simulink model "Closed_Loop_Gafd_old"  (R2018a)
settings: Solver=ode45  StartTime=0.0  StopTime=50  RelTol=1e-3  EnableMultiTasking=on
InitFcn:
  | init
StopFcn:
  | pl
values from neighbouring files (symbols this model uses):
  Cyb = -0.0245    [init.m]    (also in lqr_des.m)
  Cydel = [-0.24668,0.24668, 0.47413,-0.47413,0]/100    [init.m]    (also in lqr_des.m = [-0.24668,0.24668, 0.47413,-0.47413]/100)
  Cza = -0.073    [init.m]
  Czdel = [0.51664,0.51664,0.60478,0.60478,0.06]/100    [init.m]
  d2r = pi/180    (= 0.0174532925199)    [init.m]
  Mass = 198.32    [init.m]    (also in lqr_des.m)
  Qbar = 150    [init.m]    (also in lqr_des.m)
  r2d = 180/pi    (= 57.2957795131)    [init.m]    (also in pl.m)
  Sref = 79.069    [init.m]    (also in lqr_des.m)
  V0 = 822.8    [init.m]
undefined symbols (not defined in the file or in its folder): Abfp, Aema, Afla, Ardr, Avf, Bbfp, Bema, Bfla, Brdr, Bvf, Cbfp, Cema, Cfla, Crdr, Cvf, Dbfp, Dema, Dfla, Drdr, Dvf, K4axmix, Kf1, Kf2, Kf3, Kf4, Kf6, Kgl, Kgp, wd1, wd2, wd3, wd4, wd6, wd7, wn1, wn2, wn3, wn4, wn6, wn7, zd1, zd2, zd3, zd4, zd6, zd7, zn1, zn2, zn3, zn4, zn6, zn7

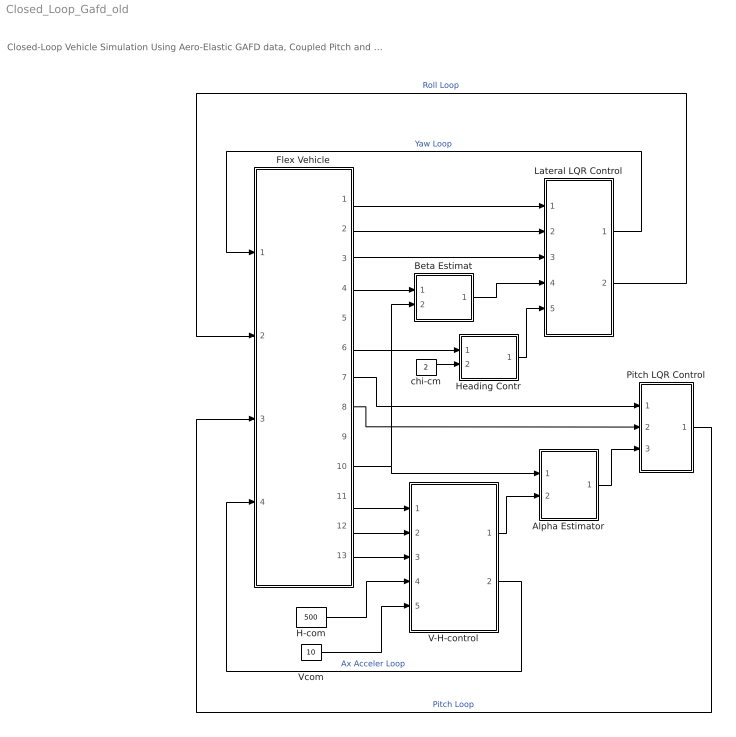
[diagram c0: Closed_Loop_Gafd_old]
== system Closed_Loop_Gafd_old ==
  note: Closed-Loop Vehicle Simulation Using Aero-Elastic GAFD data, Coupled Pitch and Lateral axes
  Alpha Estimator : Subsystem
  Beta Estimat : Subsystem
  Flex Vehicle : Subsystem
  H-com : Constant  Value=500
  Heading Contr : Subsystem
  Lateral LQR Control : Subsystem
  Pitch LQR Control : Subsystem
  V-H-control : Subsystem
  Vcom : Constant  Value=10
  chi-cm : Constant  Value=2
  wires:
  chi-cm/1 -> Heading Contr/2(chi-cmd)
  Flex Vehicle/2(p) -> Lateral LQR Control/2(p)
  Flex Vehicle/3(r) -> Lateral LQR Control/3(r)
  Flex Vehicle/1(phi) -> Lateral LQR Control/1(phi)
  Flex Vehicle/4(Ny) -> Beta Estimat/1(Ydd)
  Flex Vehicle/6("chi ") -> Heading Contr/1(chi)
  Flex Vehicle/12(Nz) -> V-H-control/2(Az)
  Flex Vehicle/13(dH) -> V-H-control/3(dH)
  Flex Vehicle/11(V-dot) -> V-H-control/1(Vdot)
  Flex Vehicle/10(delt) -> Alpha Estimator/1(delta), Beta Estimat/2(delta)
  Alpha Estimator/1(alphat) -> Pitch LQR Control/3(alfa)
  V-H-control/1(Zdd-com) -> Alpha Estimator/2(Zdd)
  Pitch LQR Control/1(elev) -> Flex Vehicle/3(ptch)  "Pitch Loop"
  Beta Estimat/1(bethat) -> Lateral LQR Control/4(bet)
  Lateral LQR Control/2(Rud) -> Flex Vehicle/2(yaw)  "Roll Loop"
  Lateral LQR Control/1(Ailer) -> Flex Vehicle/1(roll)  "Yaw Loop"
  V-H-control/2(Throtle) -> Flex Vehicle/4(Ax-cmd)  "Ax Acceler Loop"
  Flex Vehicle/8(q) -> Pitch LQR Control/2(q)
  Flex Vehicle/7(thet) -> Pitch LQR Control/1(thet)
  Heading Contr/1(phi-cmd) -> Lateral LQR Control/5(ph-cmd)
  H-com/1 -> V-H-control/4(H-comd)
  Vcom/1 -> V-H-control/5(Vcomd)

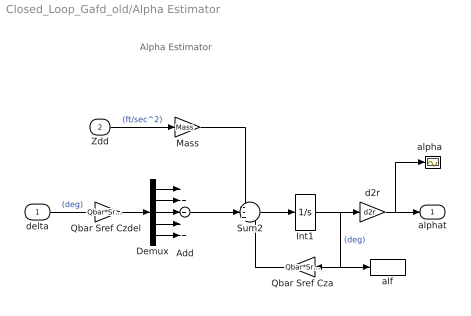
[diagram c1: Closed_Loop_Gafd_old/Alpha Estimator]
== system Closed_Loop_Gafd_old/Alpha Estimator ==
  note: Alpha Estimator
  delta : Inport
  Zdd : Inport  Port=2
  Add : Sum  Inputs=+++++
  Demux : Demux  Outputs=5
  Int1 : Integrator
  Mass : Gain  Gain=Mass
  Qbar Sref Cza : Gain  Gain=Qbar*Sref*Cza
  "Qbar Sref Czdel " : Gain  Gain=Qbar*Sref*Czdel
  Sum2 : Sum  Inputs=--+
  alf : ToWorkspace  VariableName=alphat  SampleTime=-1
  "alpha  " : Scope
  d2r : Gain  Gain=d2r
  alphat : Outport
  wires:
  Demux/5 -> Add/5
  Demux/4 -> Add/4
  Demux/3 -> Add/3
  Demux/2 -> Add/2
  Demux/1 -> Add/1
  "Qbar Sref Czdel "/1 -> Demux/1
  delta/1 -> "Qbar Sref Czdel "/1  "(deg)"
  Sum2/1 -> Int1/1
  Int1/1 -> d2r/1, Qbar Sref Cza/1, alf/1  "(deg)"
  Qbar Sref Cza/1 -> Sum2/3
  Zdd/1 -> Mass/1  "(ft/sec^2)"
  Mass/1 -> Sum2/1
  d2r/1 -> "alpha  "/1, alphat/1
  Add/1 -> Sum2/2

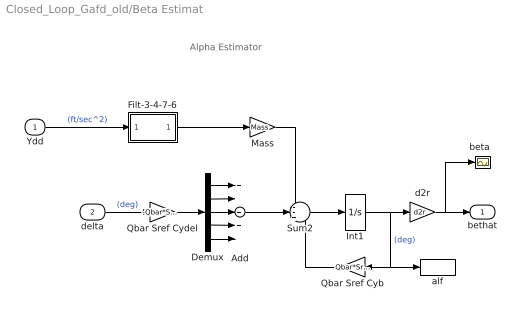
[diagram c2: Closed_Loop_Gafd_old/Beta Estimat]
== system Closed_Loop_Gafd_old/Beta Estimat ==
  note: Alpha Estimator
  Ydd : Inport
  delta : Inport  Port=2
  Add : Sum  Inputs=+++++
  Demux : Demux  Outputs=5
  Filt-3-4-7-6 : Subsystem
  Int1 : Integrator
  Mass : Gain  Gain=Mass
  Qbar Sref Cyb : Gain  Gain=Qbar*Sref*Cyb
  Qbar Sref Cydel : Gain  Gain=-Qbar*Sref*Cydel
  Sum2 : Sum  Inputs=--+
  alf : ToWorkspace  VariableName=bethat  SampleTime=-1
  "beta  " : Scope
  d2r : Gain  Gain=d2r
  bethat : Outport
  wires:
  Filt-3-4-7-6/1(Ot) -> Mass/1
  Demux/5 -> Add/5
  Demux/4 -> Add/4
  Demux/3 -> Add/3
  Demux/2 -> Add/2
  Demux/1 -> Add/1
  Qbar Sref Cydel/1 -> Demux/1
  delta/1 -> Qbar Sref Cydel/1  "(deg)"
  Sum2/1 -> Int1/1
  Int1/1 -> d2r/1, Qbar Sref Cyb/1, alf/1  "(deg)"
  Qbar Sref Cyb/1 -> Sum2/3
  Ydd/1 -> Filt-3-4-7-6/1(In)  "(ft/sec^2)"
  Mass/1 -> Sum2/1
  d2r/1 -> "beta  "/1, bethat/1
  Add/1 -> Sum2/2

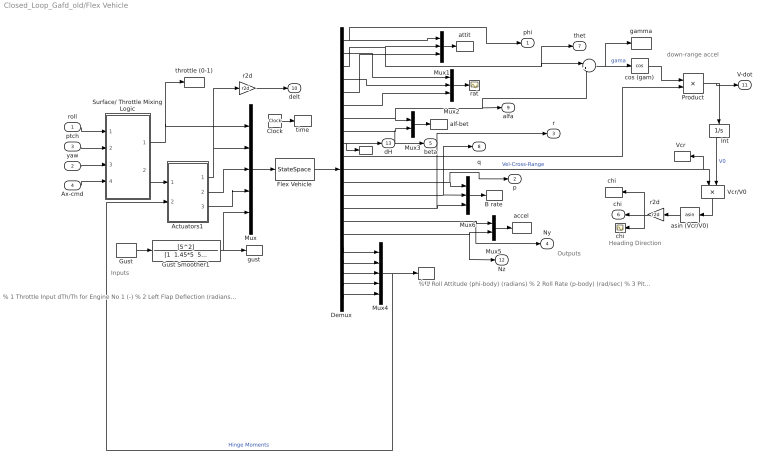
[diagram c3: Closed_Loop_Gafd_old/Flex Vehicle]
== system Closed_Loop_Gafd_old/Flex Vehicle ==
  note: % 1 Roll Attitude (phi-body) (radians) % 2 Roll Rate (p-body) (rad/sec) % 3 Pitch Attitude (thet-bdy) (radians) % 4 Pitch Rate (q-body) (rad/sec) % 5 Yaw Attitude (psi-body) (radians) % 6 Yaw Rate (r-body) (rad/sec) % 7 Angle of attack, alfa, (radians) % 8 Angle of sideslip, beta, (radian) % 9 Change in Altitude, delta-h, (feet) % 10 Forward Acceleration (V-dot) (ft/sec) % 11 Cross Range Velocity (Vcr) (ft/sec) % 12 Rate-Gyro # 1, Roll Rate (Body) (rad/sec) % 13 Rate-Gyro # 2, Pitch Rate (Body) (rad/sec) % 14 Rate-Gyro # 3, Yaw Rate (Body) (rad/sec) % 15 Accelerom # 1, (along Y), (ft/sec^2) Translat. Acceler % 16 Accelerom # 2, (along Z), (ft/sec^2) Translat. Acceler % 17 Hinge Moment for Aero Surface # 1, (ft-lb) % 18 Hinge Moment for Aero Surface # 2, (ft-lb) % 19 Hinge Moment for Aero Surface # 3, (ft-lb) % 20 Hinge Moment for Aero Surface # 4, (ft-lb) % 21 Hinge Moment for Aero Surface # 5, (ft-lb)
  note: % 1 Throttle Input dTh/Th for Engine No 1 (-) % 2 Left Flap Deflection (radians) % 3 Right Flap Deflection (radians) % 4 Left Rudder Deflection (radians) % 5 Right Rudder Deflection (radians) % 6 Body Flap Deflection (radians) % 7 Left Flap Velocity (rad/sec) % 8 Right Flap Velocity (rad/sec) % 9 Left Rudder Velocity (rad/sec) % 10 Right Rudder Velocity (rad/sec) % 11 Body Flap Velocity (rad/sec) % 12 Left Flap Acceleration (rad/s^2) % 13 Right Flap Acceleration (rad/s^2) % 14 Left Rudder Acceleration (rad/s^2) % 15 Right Rudder Acceleration (rad/s^2) % 16 Body Flap Acceleration (rad/s^2) % 17 Wind Gust Azim, Elev Angles=(45.0 90.0) (deg)
  note: Heading Direction
  note: down-range accel
  note: Inputs
  note: Outputs
  roll : Inport
  yaw : Inport  Port=2
  ptch : Inport  Port=3
  Ax-cmd : Inport  Port=4
  " " : ToWorkspace  VariableName=dH  SampleTime=-1
  "    " : Sum  Inputs=|+-
  Actuators1 : Subsystem
  B rate : ToWorkspace  VariableName=Wb  SampleTime=-1
  Clock : Clock
  Demux : Demux  Outputs=21
  Flex Vehicle : StateSpace  A=Avf  B=Bvf  C=Cvf  D=Dvf  InitialCondition=0
  Gust : DiscretePulseGenerator  PulseType=Time based  Amplitude=80  Period=100  PulseWidth=0.5  PhaseDelay=5
  Gust Smoother1 : TransferFcn  Numerator=[5^2]  Denominator="[1  1.45*5  5^2]"
  Int : Integrator  InitialCondition=V0
  Mux : Mux  Inputs=[1, 5,5,5, 1]
  Mux1 : Mux  Inputs=3
  Mux2 : Mux  Inputs=3
  Mux3 : Mux  Inputs=2
  Mux4 : Mux  Inputs=5
  Mux5 : Mux  Inputs=2
  Mux6 : Mux  Inputs=3
  Product : Product
  Surface/ Throttle Mixing Logic : Subsystem
  "Vcr " : ToWorkspace  VariableName=Vcr  SampleTime=-1
  Vcr/V0 : Product  Inputs=*/
  accel : ToWorkspace  VariableName=Accel  SampleTime=-1
  alf-bet : ToWorkspace  VariableName=albe  SampleTime=-1
  asin (Vcr/V0) : Trigonometry  Operator=asin
  attit : ToWorkspace  VariableName=attit  SampleTime=-1
  chi : Scope
  "chi  " : ToWorkspace  VariableName=chi  SampleTime=-1
  cos (gam) : Trigonometry  Operator=cos
  gamma : ToWorkspace  VariableName=gama  SampleTime=-1
  gust : ToWorkspace  VariableName=gust  SampleTime=-1
  hm : ToWorkspace  VariableName=HM  SampleTime=-1
  r2d : Gain  Gain=r2d
  "r2d " : Gain  Gain=r2d
  rat : Scope
  throttle (0-1) : ToWorkspace  VariableName=Thro  SampleTime=-1
  time : ToWorkspace  VariableName=time  SampleTime=-1
  phi : Outport
  p : Outport  Port=2
  r : Outport  Port=3
  Ny : Outport  Port=4
  beta : Outport  Port=5
  "chi " : Outport  Port=6
  thet : Outport  Port=7
  q : Outport  Port=8
  alfa : Outport  Port=9
  delt : Outport  Port=10
  V-dot : Outport  Port=11
  Nz : Outport  Port=12
  dH : Outport  Port=13
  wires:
  Mux4/1 -> Actuators1/2(HM), hm/1  "Hinge Moments"
  Demux/11 -> Vcr/V0/1, "Vcr "/1  "Vel-Cross-Range"
  Demux/9 -> dH/1, " "/1
  Demux/12 -> Mux6/1, p/1
  Demux/13 -> Mux6/2, q/1
  Demux/14 -> Mux6/3, r/1
  Demux/15 -> Mux5/1, Ny/1
  Demux/16 -> Mux5/2, Nz/1
  Demux/17 -> Mux4/1
  Demux/18 -> Mux4/2
  Demux/19 -> Mux4/3
  Demux/20 -> Mux4/4
  Demux/21 -> Mux4/5
  Demux/8 -> Mux3/2, beta/1
  Demux/7 -> Mux3/1, alfa/1, "    "/2
  Demux/2 -> Mux2/1
  Demux/6 -> Mux2/3
  Demux/5 -> Mux1/3
  Demux/3 -> Mux1/2, "    "/1, thet/1
  Demux/1 -> Mux1/1, phi/1
  Mux/1 -> Flex Vehicle/1
  Flex Vehicle/1 -> Demux/1
  Surface/ Throttle Mixing Logic/1(Thro) -> Mux/1, throttle (0-1)/1
  roll/1 -> Surface/ Throttle Mixing Logic/1(roll)
  ptch/1 -> Surface/ Throttle Mixing Logic/2(ptch)
  yaw/1 -> Surface/ Throttle Mixing Logic/3(yaw)
  Ax-cmd/1 -> Surface/ Throttle Mixing Logic/4(Ax)
  Demux/4 -> Mux2/2
  Mux1/1 -> attit/1
  Mux2/1 -> rat/1
  Mux5/1 -> accel/1
  Mux6/1 -> B rate/1
  Mux3/1 -> alf-bet/1
  r2d/1 -> delt/1
  "r2d "/1 -> "chi "/1, chi/1, "chi  "/1
  Vcr/V0/1 -> asin (Vcr/V0)/1
  asin (Vcr/V0)/1 -> "r2d "/1
  cos (gam)/1 -> Product/1
  Product/1 -> V-dot/1, Int/1
  Int/1 -> Vcr/V0/2  "V0"
  "    "/1 -> cos (gam)/1, gamma/1  "gama"
  Demux/10 -> Product/2
  Surface/ Throttle Mixing Logic/2(delta) -> Actuators1/1(del-cmd)
  Actuators1/1(delta) -> Mux/2, r2d/1
  Actuators1/2(del-dot) -> Mux/3
  Gust Smoother1/1 -> gust/1, Mux/5
  Clock/1 -> time/1
  Gust/1 -> Gust Smoother1/1
  Actuators1/3(del-ddot) -> Mux/4

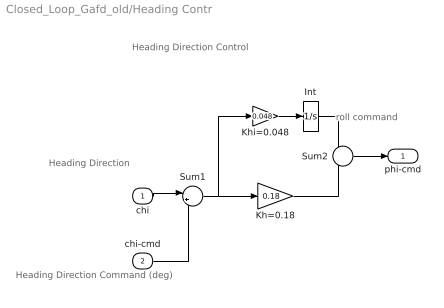
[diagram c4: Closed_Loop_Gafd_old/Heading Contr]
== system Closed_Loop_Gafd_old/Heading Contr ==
  note: Heading Direction Control
  note: Heading Direction
  note: roll command
  note: Heading Direction Command (deg)
  chi : Inport
  chi-cmd : Inport  Port=2
  Int : Integrator
  Kh=0.18 : Gain  Gain=0.18
  Khi=0.048 : Gain  Gain=0.048
  Sum1 : Sum  Inputs=|+-
  Sum2 : Sum  Inputs=--
  phi-cmd : Outport
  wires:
  Khi=0.048/1 -> Int/1
  Kh=0.18/1 -> Sum2/2
  Int/1 -> Sum2/1
  Sum2/1 -> phi-cmd/1
  Sum1/1 -> Kh=0.18/1, Khi=0.048/1
  chi/1 -> Sum1/1
  chi-cmd/1 -> Sum1/2

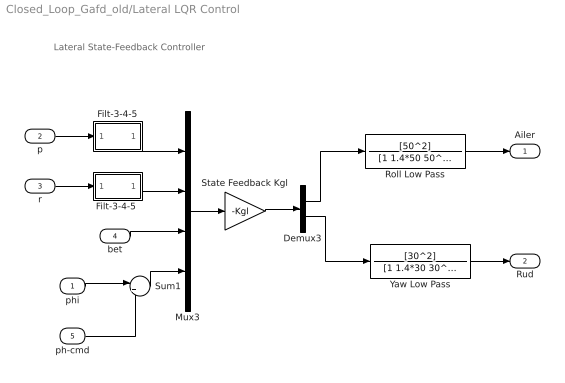
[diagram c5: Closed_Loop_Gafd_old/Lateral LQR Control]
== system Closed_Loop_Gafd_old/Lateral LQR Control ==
  note: Lateral State-Feedback Controller
  phi : Inport
  p : Inport  Port=2
  r : Inport  Port=3
  bet : Inport  Port=4
  ph-cmd : Inport  Port=5
  Demux3 : Demux  Outputs=2
  Filt-3-4-5 : Subsystem
  "Filt-3-4-5 " : Subsystem
  Mux3 : Mux
  Roll Low Pass : TransferFcn  Numerator=[50^2]  Denominator=[1 1.4*50 50^2]
  State Feedback Kgl : Gain  Gain=-Kgl  Multiplication=Matrix(K*u) (u vector)
  Sum1 : Sum  Inputs=|+-
  Yaw Low Pass : TransferFcn  Numerator=[30^2]  Denominator=[1 1.4*30 30^2]
  Ailer : Outport
  Rud : Outport  Port=2
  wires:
  Roll Low Pass/1 -> Ailer/1
  Yaw Low Pass/1 -> Rud/1
  "Filt-3-4-5 "/1(Ot) -> Mux3/2
  Filt-3-4-5/1(Ot) -> Mux3/1
  ph-cmd/1 -> Sum1/2
  phi/1 -> Sum1/1
  Sum1/1 -> Mux3/4
  Demux3/2 -> Yaw Low Pass/1
  Demux3/1 -> Roll Low Pass/1
  bet/1 -> Mux3/3
  r/1 -> "Filt-3-4-5 "/1(In)
  p/1 -> Filt-3-4-5/1(In)
  Mux3/1 -> State Feedback Kgl/1
  State Feedback Kgl/1 -> Demux3/1

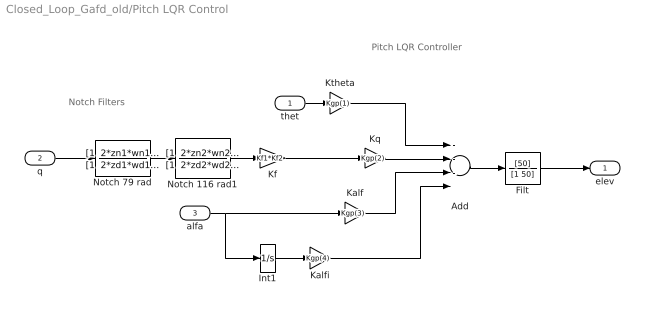
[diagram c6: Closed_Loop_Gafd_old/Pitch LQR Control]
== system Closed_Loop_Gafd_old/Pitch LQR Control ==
  note: Notch Filters
  note: Pitch LQR Controller
  thet : Inport
  q : Inport  Port=2
  alfa : Inport  Port=3
  Add : Sum  Inputs=----
  Filt : TransferFcn  Numerator=[50]  Denominator=[1 50]
  Int1 : Integrator
  Kalf : Gain  Gain=Kgp(3)
  Kalfi : Gain  Gain=Kgp(4)
  Kf : Gain  Gain=Kf1*Kf2
  Kq : Gain  Gain=Kgp(2)
  Ktheta : Gain  Gain=Kgp(1)
  Notch 116 rad1 : TransferFcn  Numerator="[1  2*zn2*wn2  wn2^2]"  Denominator="[1  2*zd2*wd2  wd2^2]"
  Notch 79 rad : TransferFcn  Numerator="[1  2*zn1*wn1  wn1^2]"  Denominator="[1  2*zd1*wd1  wd1^2]"
  elev : Outport
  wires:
  Filt/1 -> elev/1
  thet/1 -> Ktheta/1
  alfa/1 -> Kalf/1, Int1/1
  Kalf/1 -> Add/3
  Kalfi/1 -> Add/4
  Int1/1 -> Kalfi/1
  Kq/1 -> Add/2
  Ktheta/1 -> Add/1
  Add/1 -> Filt/1
  Notch 116 rad1/1 -> Kf/1
  Notch 79 rad/1 -> Notch 116 rad1/1
  Kf/1 -> Kq/1
  q/1 -> Notch 79 rad/1

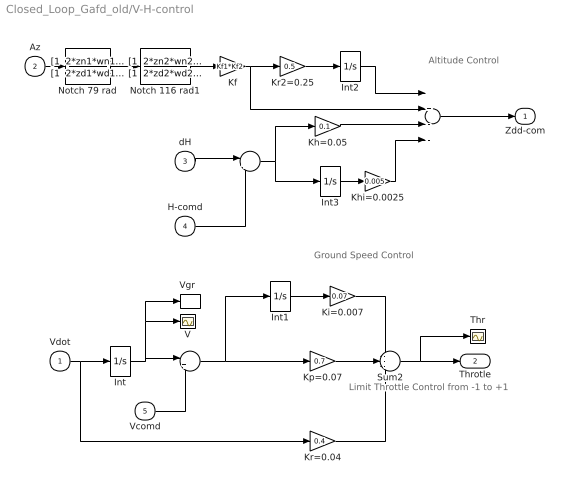
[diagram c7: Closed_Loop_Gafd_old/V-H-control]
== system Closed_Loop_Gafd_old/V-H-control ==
  note: Altitude Control
  note: Ground Speed Control
  note: Limit Throttle Control from -1 to +1
  Vdot : Inport
  Az : Inport  Port=2
  dH : Inport  Port=3
  H-comd : Inport  Port=4
  Vcomd : Inport  Port=5
  " " : Sum  Inputs=|+-
  "  " : Sum  Inputs=++--
  "    " : Sum  Inputs=|+-
  Int{,1..3} (4 alike) : Integrator
  Kf : Gain  Gain=Kf1*Kf2
  Kh=0.05 : Gain  Gain=0.1
  Khi=0.0025 : Gain  Gain=0.005
  Ki=0.007 : Gain  Gain=0.07
  Kp=0.07 : Gain  Gain=0.7
  Kr2=0.25 : Gain  Gain=0.5
  Kr=0.04 : Gain  Gain=0.4
  Notch 116 rad1 : TransferFcn  Numerator="[1  2*zn2*wn2  wn2^2]"  Denominator="[1  2*zd2*wd2  wd2^2]"
  Notch 79 rad : TransferFcn  Numerator="[1  2*zn1*wn1  wn1^2]"  Denominator="[1  2*zd1*wd1  wd1^2]"
  Sum2 : Sum  Inputs=---
  Thr : Scope
  V : Scope
  "Vgr  " : ToWorkspace  VariableName=Vgr  SampleTime=-1
  Zdd-com : Outport
  Throtle : Outport  Port=2
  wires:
  Khi=0.0025/1 -> "  "/4
  Int3/1 -> Khi=0.0025/1
  " "/1 -> Int3/1, Kh=0.05/1
  "  "/1 -> Zdd-com/1
  Az/1 -> Notch 79 rad/1
  Int2/1 -> "  "/1
  Kr2=0.25/1 -> Int2/1
  Kh=0.05/1 -> "  "/3
  H-comd/1 -> " "/2
  dH/1 -> " "/1
  Vcomd/1 -> "    "/2
  "    "/1 -> Int1/1, Kp=0.07/1
  Int/1 -> "    "/1, V/1, "Vgr  "/1
  Int1/1 -> Ki=0.007/1
  Ki=0.007/1 -> Sum2/1
  Kp=0.07/1 -> Sum2/2
  Kr=0.04/1 -> Sum2/3
  Sum2/1 -> Thr/1, Throtle/1
  Vdot/1 -> Kr=0.04/1, Int/1
  Notch 79 rad/1 -> Notch 116 rad1/1
  Notch 116 rad1/1 -> Kf/1
  Kf/1 -> "  "/2, Kr2=0.25/1

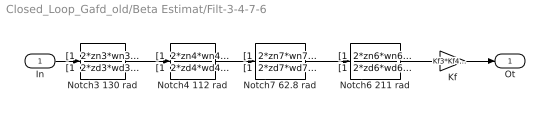
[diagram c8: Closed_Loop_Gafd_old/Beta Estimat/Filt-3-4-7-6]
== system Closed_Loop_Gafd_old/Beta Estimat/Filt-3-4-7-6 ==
  In : Inport
  Kf : Gain  Gain=Kf3*Kf4*Kf6
  Notch3 130 rad : TransferFcn  Numerator="[1  2*zn3*wn3  wn3^2]"  Denominator="[1  2*zd3*wd3  wd3^2]"
  Notch4 112 rad : TransferFcn  Numerator="[1  2*zn4*wn4  wn4^2]"  Denominator="[1  2*zd4*wd4  wd4^2]"
  Notch6 211 rad : TransferFcn  Numerator="[1  2*zn6*wn6  wn6^2]"  Denominator="[1  2*zd6*wd6  wd6^2]"
  Notch7 62.8 rad : TransferFcn  Numerator="[1  2*zn7*wn7  wn7^2]"  Denominator="[1  2*zd7*wd7  wd7^2]"
  Ot : Outport
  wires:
  Notch7 62.8 rad/1 -> Notch6 211 rad/1
  Kf/1 -> Ot/1
  Notch6 211 rad/1 -> Kf/1
  In/1 -> Notch3 130 rad/1
  Notch3 130 rad/1 -> Notch4 112 rad/1
  Notch4 112 rad/1 -> Notch7 62.8 rad/1

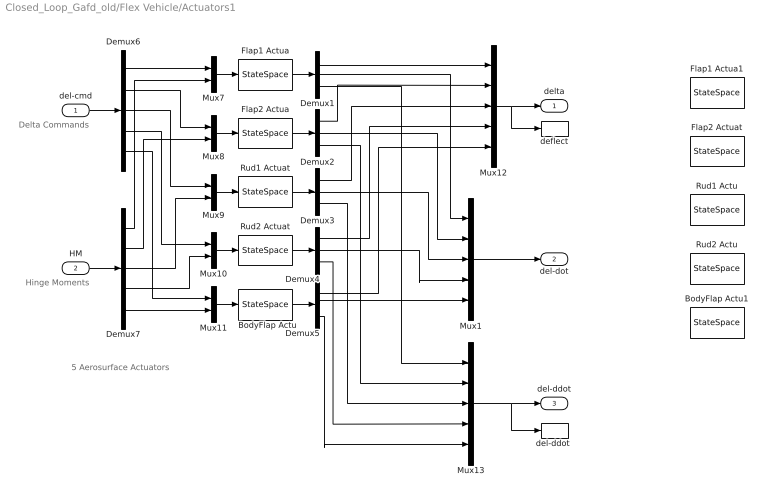
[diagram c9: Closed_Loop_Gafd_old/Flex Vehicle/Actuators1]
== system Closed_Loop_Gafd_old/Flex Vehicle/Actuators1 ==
  note: 5 Aerosurface Actuators
  note: Hinge Moments
  note: Delta Commands
  del-cmd : Inport
  HM : Inport  Port=2
  BodyFlap Actu : StateSpace  A=Abfp  B=Bbfp  C=Cbfp  D=Dbfp  InitialCondition=0
  BodyFlap Actu1 : StateSpace  A=Aema  B=Bema  C=Cema  D=Dema  InitialCondition=0
  Demux{1..5} (5 alike) : Demux  Outputs=3
  Demux6 : Demux  Outputs=5
  Demux7 : Demux  Outputs=5
  Flap1 Actua : StateSpace  A=Afla  B=Bfla  C=Cfla  D=Dfla  InitialCondition=0
  Flap1 Actua1 : StateSpace  A=Aema  B=Bema  C=Cema  D=Dema  InitialCondition=0
  Flap2 Actua : StateSpace  A=Afla  B=Bfla  C=Cfla  D=Dfla  InitialCondition=0
  Flap2 Actuat : StateSpace  A=Aema  B=Bema  C=Cema  D=Dema  InitialCondition=0
  Mux1 : Mux  Inputs=5
  Mux{7..11} (5 alike) : Mux  Inputs=2
  Mux12 : Mux  Inputs=5
  Mux13 : Mux  Inputs=5
  Rud1 Actu : StateSpace  A=Aema  B=Bema  C=Cema  D=Dema  InitialCondition=0
  Rud1 Actuat : StateSpace  A=Ardr  B=Brdr  C=Crdr  D=Drdr  InitialCondition=0
  Rud2 Actu : StateSpace  A=Aema  B=Bema  C=Cema  D=Dema  InitialCondition=0
  Rud2 Actuat : StateSpace  A=Ardr  B=Brdr  C=Crdr  D=Drdr  InitialCondition=0
  deflect : ToWorkspace  VariableName=delta  SampleTime=-1
  "del-ddot " : ToWorkspace  VariableName=deldd  SampleTime=-1
  delta : Outport
  del-dot : Outport  Port=2
  del-ddot : Outport  Port=3
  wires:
  Mux7/1 -> Flap1 Actua/1
  Flap1 Actua/1 -> Demux1/1
  Mux8/1 -> Flap2 Actua/1
  Flap2 Actua/1 -> Demux2/1
  Mux9/1 -> Rud1 Actuat/1
  Rud1 Actuat/1 -> Demux3/1
  Mux10/1 -> Rud2 Actuat/1
  Rud2 Actuat/1 -> Demux4/1
  Mux11/1 -> BodyFlap Actu/1
  BodyFlap Actu/1 -> Demux5/1
  Demux6/1 -> Mux7/1
  Demux6/2 -> Mux8/1
  Demux6/3 -> Mux9/1
  Demux6/4 -> Mux10/1
  Demux6/5 -> Mux11/1
  Demux7/5 -> Mux11/2
  Demux7/4 -> Mux10/2
  Demux7/3 -> Mux9/2
  Demux7/2 -> Mux8/2
  Demux7/1 -> Mux7/2
  Demux1/1 -> Mux12/1
  Demux2/1 -> Mux12/2
  Demux3/1 -> Mux12/3
  Demux4/1 -> Mux12/4
  Demux5/1 -> Mux12/5
  Demux4/3 -> Mux13/4
  Demux3/3 -> Mux13/3
  Demux2/3 -> Mux13/2
  Demux1/3 -> Mux13/1
  Demux1/2 -> Mux1/1
  Mux12/1 -> deflect/1, delta/1
  del-cmd/1 -> Demux6/1
  Demux2/2 -> Mux1/2
  Demux3/2 -> Mux1/3
  Demux4/2 -> Mux1/4
  HM/1 -> Demux7/1
  Mux13/1 -> "del-ddot "/1, del-ddot/1
  Demux5/2 -> Mux1/5
  Demux5/3 -> Mux13/5
  Mux1/1 -> del-dot/1

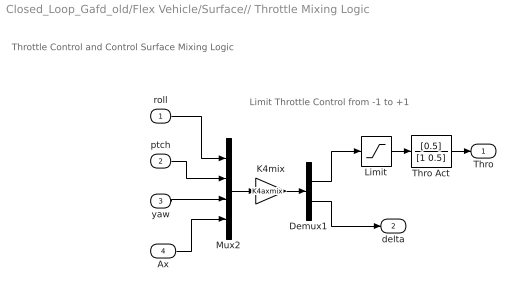
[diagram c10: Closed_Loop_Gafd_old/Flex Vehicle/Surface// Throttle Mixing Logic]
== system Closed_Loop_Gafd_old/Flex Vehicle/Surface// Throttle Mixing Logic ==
  note: Limit Throttle Control from -1 to +1
  note: Throttle Control and Control Surface Mixing Logic
  roll : Inport
  ptch : Inport  Port=2
  yaw : Inport  Port=3
  Ax : Inport  Port=4
  Demux1 : Demux  Outputs=[1, 5]
  K4mix : Gain  Gain=K4axmix  Multiplication=Matrix(K*u) (u vector)
  Limit : Saturate  UpperLimit=1  LowerLimit=-1
  Mux2 : Mux
  Thro Act : TransferFcn  Numerator=[0.5]  Denominator=[1 0.5]
  Thro : Outport
  delta : Outport  Port=2
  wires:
  Thro Act/1 -> Thro/1
  Limit/1 -> Thro Act/1
  K4mix/1 -> Demux1/1
  Mux2/1 -> K4mix/1
  Demux1/1 -> Limit/1
  Demux1/2 -> delta/1
  roll/1 -> Mux2/1
  Ax/1 -> Mux2/4
  yaw/1 -> Mux2/3
  ptch/1 -> Mux2/2

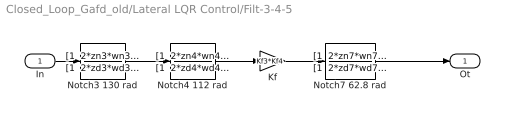
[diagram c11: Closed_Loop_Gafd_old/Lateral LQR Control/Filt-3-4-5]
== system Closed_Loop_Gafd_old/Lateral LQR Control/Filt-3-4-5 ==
  In : Inport
  Kf : Gain  Gain=Kf3*Kf4
  Notch3 130 rad : TransferFcn  Numerator="[1  2*zn3*wn3  wn3^2]"  Denominator="[1  2*zd3*wd3  wd3^2]"
  Notch4 112 rad : TransferFcn  Numerator="[1  2*zn4*wn4  wn4^2]"  Denominator="[1  2*zd4*wd4  wd4^2]"
  Notch7 62.8 rad : TransferFcn  Numerator="[1  2*zn7*wn7  wn7^2]"  Denominator="[1  2*zd7*wd7  wd7^2]"
  Ot : Outport
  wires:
  Notch7 62.8 rad/1 -> Ot/1
  In/1 -> Notch3 130 rad/1
  Kf/1 -> Notch7 62.8 rad/1
  Notch3 130 rad/1 -> Notch4 112 rad/1
  Notch4 112 rad/1 -> Kf/1

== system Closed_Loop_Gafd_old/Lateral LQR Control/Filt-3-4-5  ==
  In : Inport
  Kf : Gain  Gain=Kf3*Kf4
  Notch3 130 rad : TransferFcn  Numerator="[1  2*zn3*wn3  wn3^2]"  Denominator="[1  2*zd3*wd3  wd3^2]"
  Notch4 112 rad : TransferFcn  Numerator="[1  2*zn4*wn4  wn4^2]"  Denominator="[1  2*zd4*wd4  wd4^2]"
  Notch7 62.8 rad : TransferFcn  Numerator="[1  2*zn7*wn7  wn7^2]"  Denominator="[1  2*zd7*wd7  wd7^2]"
  Ot : Outport
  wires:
  Notch7 62.8 rad/1 -> Ot/1
  In/1 -> Notch3 130 rad/1
  Kf/1 -> Notch7 62.8 rad/1
  Notch3 130 rad/1 -> Notch4 112 rad/1
  Notch4 112 rad/1 -> Kf/1
